PROGRAM MAIN
VAR
    sendToB : BOOL := FALSE; // HMI can set this

    A_DataToSend   : ST_A_To_B;
    B_DataReceived : ST_B_To_A; // PLC B writes into this variable by ADS

    SendTimer      : TON;
    OneMinutePulse : BOOL;
    SeqA           : UDINT;

    CommsSendToB   : FB_AdsSend_A_To_B;

    SendBusy       : BOOL;
    SendDone       : BOOL;
    SendError      : BOOL;
    SendErrId      : UDINT;
END_VAR

SendTimer(IN := NOT SendTimer.Q, PT := T#30s);
OneMinutePulse := SendTimer.Q;

IF OneMinutePulse AND sendToB THEN
    SeqA := SeqA + 1;
    A_DataToSend.SequenceNo := SeqA;
    A_DataToSend.StartCmd   := TRUE;
    A_DataToSend.Setpoint   := 123.45 +  UDINT_TO_REAL(SeqA);
    A_DataToSend.Mode       := 1;		
	A_DataToSend.HelloFromA := CONCAT(
    'Hello from A to B  with Sequence ',
    UDINT_TO_STRING(A_DataToSend.SequenceNo)
);
END_IF

CommsSendToB(
    xExecute       := OneMinutePulse AND sendToB,
    sRemoteNetId   := '10.10.1.84.1.1',
    nRemoteAdsPort := 851,
    sRemoteSymbol  := 'MAIN.A_DataReceived',
    stData         := A_DataToSend,
    xBusy          => SendBusy,
    xDone          => SendDone,
    xError         => SendError,
    nErrId         => SendErrId
);

END_PROGRAM
